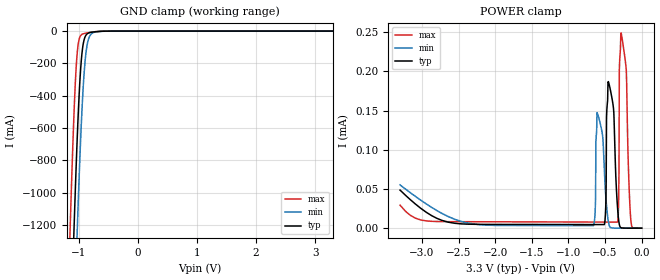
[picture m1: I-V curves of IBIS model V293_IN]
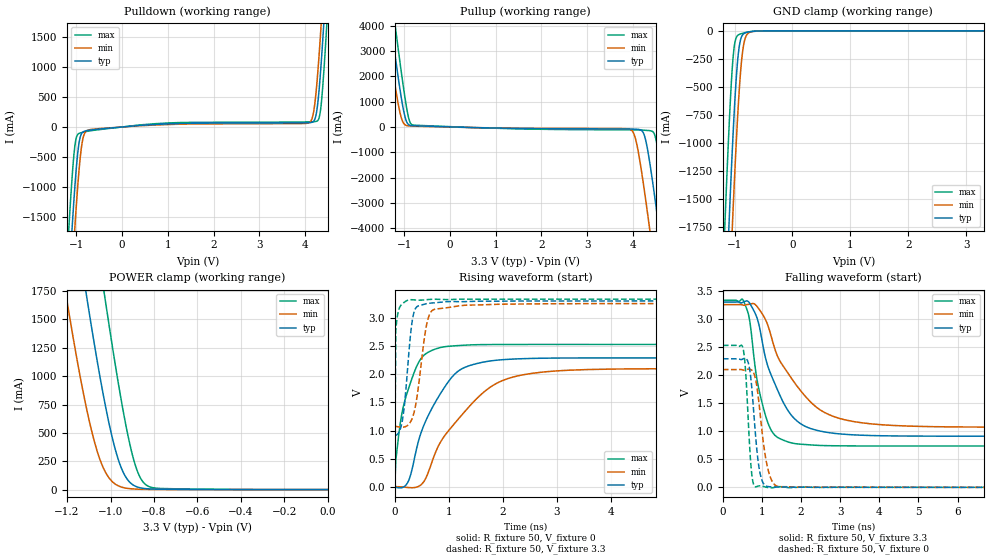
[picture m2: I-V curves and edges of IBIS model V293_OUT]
| TEXAS INSTRUMENTS INCORPORATED
| Standard Linear and Logic Group
| IBIS Model of SN74V293
| High Frequency Low voltage FIFO
| This file contains package information for the following:
|  U*BGA 100-pin (GGM) package as [Component] V293_GGM
|  TQFP 80-pin (PZA)package as [Component] V293_PZA
| This device can be powered at the following Vccs:
|  3.3 volt Vcc
| This file provides unique models under the [Model Selector] for each Vcc.
| For operation at a specific Vcc, select the appropriate model after each
| [Model Selector] keyword.
[IBIS Ver]   3.2
[Comment char]  |_char
[File Name]   sn74v293.ibs
[File Rev]   1.1 | x
[Date]   November 2, 2006
[Source]   Data created from TI-SPICE simulations at TI-SLL.
[Notes]   The following is an IBIS list for the V293.
   Please contact sllibis@ti.com with questions and
   comments concerning SLL IBIS models.
   Release 1.1 - Small tweaks for rising waveforms and saving in
   non-octet format for ease of download.
[Disclaimer] Property of Texas Instruments Incorporated.  Unauthorized
   reproduction and/or distribution is strictly prohibited.
   This product is protected under copyright law.
   Created  2001, (C) Copyright  2001, Texas Instruments
   Incorporated, All Rights Reserved
   UNLESS THERE IS A SIGNED, WRITTEN AGREEMENT TO THE
   CONTRARY, TEXAS INSTRUMENTS (TI) IS PROVIDING THE IBIS
   MODELS  AND WITHOUT ANY WARRANTY, EXPRESSED OR
   IMPLIED.  TI assumes no liability for:
   1) the accuracy of the IBIS models provided to your
   company;
   2) the proper functioning of these IBIS Models in your
   design or for any resulting applications; or
   3) infringement of patents, copyrights or intellectual
   property rights resulting from your use of these IBIS
   models.
   TI provides IBIS Models as a service to our customers.
   You and your company shall not distribute, sell or give
   these models to anyone else without prior written
   permission from TI.
   TI reserves the right to make changes to our products or
   to discontinue any semiconductor product or service
   without notice, and advises our customers to obtain the
   latest version of relevant information to verify, before
   placing orders, that the information being relied on is
   current.
   Please be aware that your receipt and use of the IBIS
   information provided shall serve as acceptance of these
   terms and conditions.  If you do not accept these terms,
   you should return or destroy the IBIS models and any
   other accompanying information immediately.
| Component V293_GGM 100-pin U*BGA
[Component]   V293_GGM
[Manufacturer]   Texas Instruments, Inc.
[Package]
|   typ   min   max
R_pkg   6.500e-02   3.500e-02   9.700e-02
L_pkg   1.952e-09   1.000e-09   3.191e-09
C_pkg   2.830e-13   1.620e-13   4.340e-13
[Pin]   signal_name   model_name   R_pin   L_pin   C_pin
9   D   V293_IN   6.000e-02   1.666e-09   2.470e-13
94   GND   GND   7.300e-02   2.168e-09   3.190e-13
95   VCC   POWER   8.600e-02   2.675e-09   3.620e-13
99   Q   V293_OUT   4.500e-02   1.418e-09   2.090e-13
| Component V293_PZA 80-pin TQFP
[Component]   V293_PZA
[Manufacturer]   Texas Instruments, Inc.
[Package]
|   typ   min   max
R_pkg   7.900e-02   6.900e-02   8.800e-02
L_pkg   3.924e-09   3.514e-09   4.476e-09
C_pkg   6.910e-13   6.420e-13   7.610e-13
[Pin]   signal_name   model_name   R_pin   L_pin   C_pin
9   D   V293_IN   6.000e-02   1.666e-09   2.470e-13
94   GND   GND   7.300e-02   2.168e-09   3.190e-13
95   VCC   POWER   8.600e-02   2.675e-09   3.620e-13
99   Q   V293_OUT   4.500e-02   1.418e-09   2.090e-13
| Models and submodels in the file (2): V293_IN (Input), V293_OUT (3-state)
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| Model V293_IN
[Model]   V293_IN
Model_type  Input
Vinl =   0.8
Vinh =   2.0
| variable   typ   min   max
C_comp   2.14pF   1.18pF   2.85pF
[Temperature Range]   40   100   -40
| Ambient temperature   25   85   -40
[Voltage range]   3.3   3.15   3.45
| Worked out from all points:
|   GND clamp passes 1 mA (typ) near -0.60 V on its own axis
[GND Clamp]
| V293_IN
|   Voltage   I(typ)   I(min)   I(max)
-3.3V     -33.46A    -34.04A    -32.82A
-1.15V    -2.039A    -2.701A    -1.248A
-1.085V   -1.256A    -1.892A    -532.2mA
-1.055V   -928.5mA   -1.54A     -283.5mA
-1.03V    -680.7mA   -1.26A     -142.6mA
-985mV    -321.5mA   -803.2mA   -38.31mA
-940mV    -113.1mA   -433.3mA   -18.76mA
-900mV    -40.32mA   -207.7mA   -14.09mA
-855mV    -15.77mA   -75.84mA   -10.85mA
-810mV    -8.755mA   -26.88mA   -8.104mA
-715mV    -3.778mA   -4.998mA   -3.386mA
3.3V      229.1pA    645.9pA    188.1pA
[POWER Clamp]
| V293_IN
|   Voltage   I(typ)   I(min)   I(max)
-3.3V     48.54uA    55.2uA     29.34uA
-660mV    4.6uA      3.184uA    7.795uA
-610mV    4.594uA    147.3uA    7.783uA
-510mV    4.603uA    75.65uA    7.758uA
-455mV    186.9uA    8.481uA    7.744uA
-330mV    26.76uA    32.16nA    7.668uA
-310mV    7.347uA    18.57nA    69.81uA
-305mV    4.736uA    16.18nA    201.7uA
-280mV    519.9nA    8.187nA    249uA
-210mV    38.91nA    1.494nA    201.5uA
-145mV    4.742nA    622.8pA    7.825uA
-48.03fV  229.1pA    487.4pA    2.678nA
| Model V293_OUT
[Model]   V293_OUT
Model_type  3-state
Enable   Active-Low
Vref =   2.0
Rref =   510
Cref =   30
Vmeas =   1.5
| variable   typ   min   max
C_comp   0.00pF   0.00pF   0.00pF
| C_pullup   3.75pF   0.81pF   8.26pF
| C_pulldown   4.76pF   0.61pF   13.29pF
[Temperature Range]   40   100   -40
| Ambient temperature   25   85   -40
[Voltage range]   3.3   3.15   3.45
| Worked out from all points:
|   slope of the pulldown table from 0 to 0.495 V, typ, clamps not added: 15.9 ohm
|   slope of the pullup table from 0 to 0.495 V, typ, clamps not added: 18.4 ohm
|   GND clamp passes 1 mA (typ) near -0.57 V on its own axis
|   POWER clamp passes 1 mA (typ) near -0.58 V on its own axis
|   rising waveform, R_fixture 50, V_fixture 0: 20-80 % time 614ps typ, 966ps min, 331ps max; typ from -0.006 V to 2.29 V
|   falling waveform, R_fixture 50, V_fixture 3.3: 20-80 % time 701ps typ, 1.08ns min, 384ps max; typ from 3.3 V to 0.911 V
|   rising waveform, R_fixture 50, V_fixture 3.3: 20-80 % time 135ps typ, 181ps min, 16.6ps max; typ from 0.908 V to 3.3 V
|   falling waveform, R_fixture 50, V_fixture 0: 20-80 % time 172ps typ, 229ps min, 119ps max; typ from 2.29 V to 0 V
[GND Clamp]
| V293_OUT
|   Voltage   I(typ)   I(min)   I(max)
-3.3V     -33.91A    -34.57A    -33.15A
-1.165V   -2.613A    -3.356A    -1.714A
-1.095V   -1.725A    -2.45A     -868.6mA
-1.035V   -1.031A    -1.716A    -307mA
-1.005V   -724.9mA   -1.372A    -142.9mA
-975mV    -462.6mA   -1.05A     -67.24mA
-920mV    -146.7mA   -543.8mA   -32.39mA
-880mV    -55.45mA   -277.8mA   -24.98mA
-840mV    -25.44mA   -118.6mA   -19.47mA
-790mV    -13.9mA    -37.1mA    -13.48mA
-725mV    -7.723mA   -10.8mA    -7.082mA
3.3V      143.7pA    790.6pA    105.6pA
[POWER Clamp]
| V293_OUT
|   Voltage   I(typ)   I(min)   I(max)
-3.3V     33.66A     32.03A     35.22A
-1.215V   3.055A     1.837A     4.273A
-1.2V     2.855A     1.659A     4.061A
-1.115V   1.765A     755.9mA    2.879A
-1.105V   1.643A     666.2mA    2.742A
-1.075V   1.288A     428.3mA    2.337A
-1.03V    801.2mA    178.4mA    1.744A
-985mV    403.2mA    58.27mA    1.182A
-945mV    166.6mA    19.81mA    726.2mA
-890mV    33.89mA    5.176mA    240mA
-840mV    8.895mA    2.135mA    46.48mA
-48.03fV  143.7pA    308.1pA    1.089nA
[Pulldown]
| V293_OUT
|   Voltage   I(typ)   I(min)   I(max)
-3.3V     -33.91A    -34.57A    -33.15A
-1.165V   -2.621A    -3.362A    -1.726A
-1.1V     -1.797A    -2.521A    -944.5mA
-1.035V   -1.048A    -1.726A    -348.3mA
-910mV    -160.7mA   -491.1mA   -99.67mA
-695mV    -51.78mA   -43.75mA   -63.64mA
4.075V    69.58mA    65.42mA    84.23mA
4.26V     283.1mA    733.1mA    96.18mA
4.355V    1.082A     1.73A      387.9mA
4.4V      1.596A     2.275A     803.2mA
4.49V     2.732A     3.433A     1.885A
6.6V      33.66A     34.27A     32.97A
[Pullup]
| V293_OUT
|   Voltage   I(typ)   I(min)   I(max)
-3.3V     33.66A     32.03A     35.22A
-1.405V   5.683A     4.305A     7.004A
-1.305V   4.285A     2.973A     5.56A
-1.195V   2.795A     1.611A     3.996A
-950mV    222.1mA    56.66mA    798.4mA
-810mV    47.21mA    31.51mA    77.2mA
3.96V     -83.05mA   -115.8mA   -115.8mA
4.23V     -244.4mA   -2.273A    -128.4mA
4.42V     -2.049A    -4.78A     -170.1mA
4.56V     -3.896A    -6.732A    -1.067A
4.78V     -6.986A    -9.877A    -3.963A
6.6V      -33.91A    -36.81A    -30.9A
[Ramp]
| V293_OUT
| variable   typ   min   max
dV/dt_r   1.38/6.14E-10   1.27/9.67E-10   1.30/3.30E-10
dV/dt_f   1.45/7.02E-10   1.32/1.08E-09   1.57/3.87E-10
R_load = 50
[Rising Waveform]
| V293_OUT
R_fixture =   50
C_fixture =   0
L_fixture =   0
V_fixture =   0
V_fixture_min = 0
V_fixture_max = 0
|   Time   V(typ)   V(min)   V(max)
0s        -5.671mV   4.55mV     90mV
15ps      -8.203mV   4.117mV    471.8mV
120ps     -16.55mV   -1.954mV   1.257V
255ps     114.9mV    -12.98mV   1.756V
360ps     499.7mV    -13.41mV   2.042V
565ps     1.158V     140.6mV    2.358V
1ns       1.879V     1.004V     2.496V
1.92ns    2.251V     1.854V     2.526V
3.23ns    2.287V     2.071V     2.528V
25ns      2.289V     2.098V     2.528V
[Falling Waveform]
| V293_OUT
R_fixture =   50
C_fixture =   0
L_fixture =   0
V_fixture =   3.3
V_fixture_min = 3.15
V_fixture_max = 3.45
|   Time   V(typ)   V(min)   V(max)
0s        3.3V       3.254V     3.332V
500ps     3.292V     3.248V     3.349V
695ps     3.268V     3.263V     2.921V
875ps     3.011V     3.219V     1.909V
1.15ns    2.155V     2.885V     1.15V
1.41ns    1.714V     2.315V     884.8mV
1.845ns   1.213V     1.851V     779.1mV
2.73ns    972.1mV    1.29V      741.7mV
4.335ns   916mV      1.103V     736.3mV
25ns      910.7mV    1.071V     736.2mV
[Rising Waveform]
| V293_OUT
R_fixture =   50
C_fixture =   0
L_fixture =   0
V_fixture =   3.3
V_fixture_min = 3.15
V_fixture_max = 3.45
|   Time   V(typ)   V(min)   V(max)
0s        907.9mV    1.074V     850mV
15ps      914.5mV    1.072V     2.777V
30ps      921.6mV    1.07V      2.925V
150ps     1.258V     1.059V     3.26V
285ps     2.672V     1.148V     3.321V
385ps     3.173V     1.462V     3.317V
550ps     3.243V     2.673V     3.319V
640ps     3.26V      3.059V     3.327V
1.29ns    3.288V     3.223V     3.332V
25ns      3.3V       3.254V     3.332V
[Falling Waveform]
| V293_OUT
R_fixture =   50
C_fixture =   0
L_fixture =   0
V_fixture =   0
V_fixture_min = 0
V_fixture_max = 0
|   Time   V(typ)   V(min)   V(max)
0s        2.289V     2.098V     2.528V
515ps     2.288V     2.091V     2.474V
585ps     2.294V     2.096V     2.019V
680ps     2.119V     2.103V     771.4mV
745ps     1.72V      2.083V     195.9mV
825ps     1.008V     1.955V     10.31mV
1.005ns   114.1mV    970.8mV    22.34mV
1.185ns   11.26mV    237.9mV    -8.012mV
1.425ns   5.987mV    12.96mV    11.74mV
25ns      -65.31nV   -66.36nV   -11.81nV
